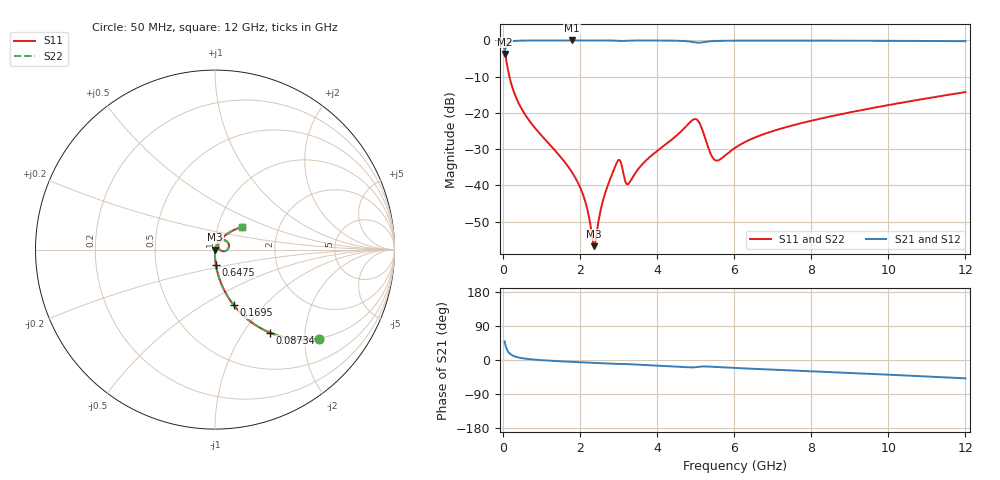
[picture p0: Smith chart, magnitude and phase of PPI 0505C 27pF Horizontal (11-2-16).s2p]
# MHz S MA R 50
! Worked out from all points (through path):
!   1601 points, 50 MHz to 12 GHz, reference 50 ohm
!   highest |S21| = -0.01 dB at 1.798 GHz (marker M1); lowest = -3.8 dB at 50 MHz (marker M2)
!   group delay of S21, straight-line fit = 12.3 ps
!   lowest |S11| = -56.7 dB at 2.373 GHz (marker M3), VSWR 1.00, Z = 50.1 - j0.0275 ohm
!   |S11| at or under -10 dB: 174.9 MHz to end of sweep
!   |S22| runs from -56.7 to -2.4 dB; largest |S21 - S12| = 0
!   S11 on the Smith chart (normalised r, x): 50 MHz: 0.99, -2.34; 87.34 MHz: 0.99, -1.34; 169.5 MHz: 0.99, -0.69; 647.5 MHz: 1.00, -0.17; 12 GHz: 1.30, +0.34
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50  0.7605 -40.6  0.6492 49.3  0.6492 49.3  0.7605 -40.6
87.34375  0.5565 -56.4  0.8305 33.5  0.8305 33.5  0.5565 -56.4
169.5  0.3253 -71.5  0.9452 18.4  0.9452 18.4  0.3253 -71.5
356.2188  0.1591 -81.8  0.9867 8.0  0.9867 8.0  0.1591 -81.8
647.5  0.08421 -86.8  0.9957 2.7  0.9957 2.7  0.08421 -86.8
1797.688  0.01521 -90.7  0.9987 -4.9  0.9987 -4.9  0.01521 -90.7
2044.156  0.008483 -87.9  0.9986 -6.1  0.9986 -6.1  0.008483 -87.9
2178.594  0.005115 -82.1  0.9986 -6.7  0.9986 -6.7  0.005115 -82.1
2372.781  0.001456 -10.9  0.9984 -7.6  0.9984 -7.6  0.001456 -10.9
2626.719  0.006928 64.3  0.9978 -8.8  0.9978 -8.8  0.006928 64.3
2970.281  0.02122 47.8  0.9885 -10.6  0.9885 -10.6  0.02122 47.8
3052.438  0.02158 25.0  0.9822 -10.5  0.9822 -10.5  0.02158 25.0
3179.406  0.01138 21.7  0.9902 -10.6  0.9902 -10.6  0.01138 21.7
3254.094  0.01047 42.0  0.9934 -10.9  0.9934 -10.9  0.01047 42.0
4038.312  0.03085 68.7  0.9957 -14.7  0.9957 -14.7  0.03085 68.7
4986.844  0.08241 25.1  0.9391 -19.3  0.9391 -19.3  0.08241 25.1
5121.281  0.06968 0.2  0.9331 -17.6  0.9331 -17.6  0.06968 0.2
5502.188  0.02249 14.2  0.9806 -18.3  0.9806 -18.3  0.02249 14.2
6025  0.03302 55.7  0.9915 -21.1  0.9915 -21.1  0.03302 55.7
8019.156  0.07845 57.3  0.9925 -29.9  0.9925 -29.9  0.07845 57.3
10013.31  0.1287 49.4  0.9871 -38.8  0.9871 -38.8  0.1287 49.4
12000  0.1939 40.2  0.9758 -48.5  0.9758 -48.5  0.1939 40.2
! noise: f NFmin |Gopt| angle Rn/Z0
50  0.000369  0.8586  0.9493  0.0005583
1372  0.003686  0.6523  4.583  0.002014
2701  0.008133  0.6844  8.657  0.00497
4031  0.01203  0.6832  12.81  0.007271
5360  0.04004  0.8609  17.13  0.06029
6682  0.01819  0.6615  21.02  0.009953
8012  0.01785  0.6039  24.78  0.007961
9341  0.01925  0.5818  28.44  0.007911
1.067e+04  0.02121  0.5736  32  0.008378
1.2e+04  0.02353  0.5734  35.47  0.009134
